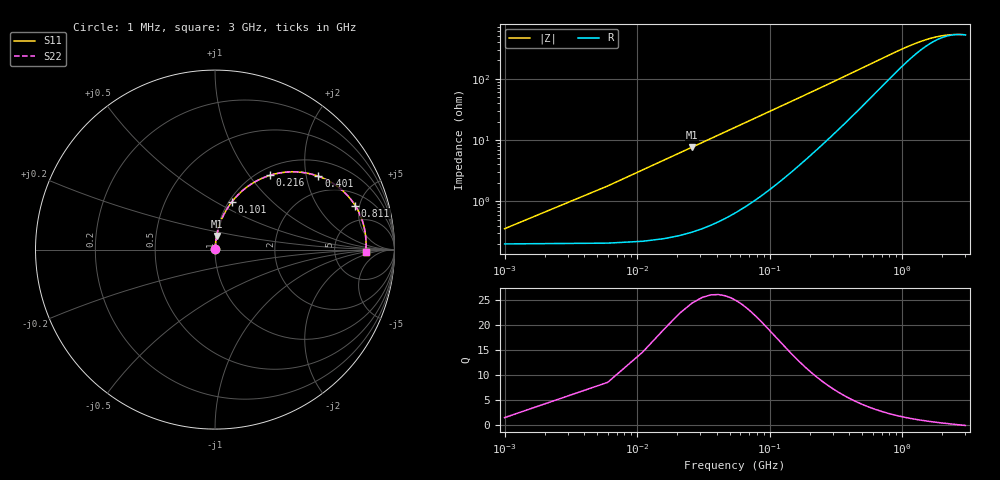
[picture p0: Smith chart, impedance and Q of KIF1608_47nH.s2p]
# MHz S RI R 50
!Freq ReS11 ImS11 ReS21 ImS21 ReS12 ImS12 ReS22 ImS22
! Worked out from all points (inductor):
!   601 points, 1 MHz to 3 GHz, reference 50 ohm
!   read as one part in series: L = 46.8 nH near 16 MHz
!   highest Q = 24.4 at 26 MHz (marker M1), where L = 46.8 nH
!   self-resonance near 2.732 GHz
!   S11 on the Smith chart (normalised r, x): 1 MHz: 1.00, +0.01; 101 MHz: 1.03, +0.59; 216 MHz: 1.13, +1.27; 401 MHz: 1.44, +2.36; 811 MHz: 3.05, +4.55; 3 GHz: 11, -1
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1  0.00202 0.00293  0.998 -0.00293  0.998 -0.00293  0.00202 0.00293
11  0.00326 0.0322  0.9967 -0.0322  0.9967 -0.0322  0.00326 0.0322
21  0.00653 0.0612  0.9935 -0.0612  0.9935 -0.0612  0.00653 0.0612
26  0.00889 0.0756  0.9911 -0.0756  0.9911 -0.0756  0.00889 0.0756
31  0.0117 0.0898  0.9883 -0.0898  0.9883 -0.0898  0.0117 0.0898
41  0.0187 0.1176  0.9813 -0.1176  0.9813 -0.1176  0.0187 0.1176
56  0.0323 0.1579  0.9677 -0.1579  0.9677 -0.1579  0.0323 0.1579
76  0.0559 0.2082  0.9441 -0.2082  0.9441 -0.2082  0.0559 0.2082
101  0.0925 0.2644  0.9075 -0.2644  0.9075 -0.2644  0.0925 0.2644
151  0.1814 0.351  0.8186 -0.351  0.8186 -0.351  0.1814 0.351
216  0.3058 0.4137  0.6942 -0.4137  0.6942 -0.4137  0.3058 0.4137
296  0.4426 0.4333  0.5574 -0.4333  0.5574 -0.4333  0.4426 0.4333
401  0.5759 0.4088  0.4241 -0.4088  0.4241 -0.4088  0.5759 0.4088
501  0.6605 0.3671  0.3395 -0.3671  0.3395 -0.3671  0.6605 0.3671
641  0.7333 0.3069  0.2667 -0.3069  0.2667 -0.3069  0.7333 0.3069
811  0.7814 0.245  0.2186 -0.245  0.2186 -0.245  0.7814 0.245
1001  0.8093 0.1917  0.1907 -0.1917  0.1907 -0.1917  0.8093 0.1917
1241  0.8266 0.142  0.1734 -0.142  0.1734 -0.142  0.8266 0.142
1501  0.8354 0.1027  0.1646 -0.1027  0.1646 -0.1027  0.8354 0.1027
2001  0.8411 0.0505  0.1589 -0.0505  0.1589 -0.0505  0.8411 0.0505
2501  0.8417 0.0139  0.1583 -0.0139  0.1583 -0.0139  0.8417 0.0139
3000  0.8403 -0.0146  0.1597 0.0146  0.1597 0.0146  0.8403 -0.0146
